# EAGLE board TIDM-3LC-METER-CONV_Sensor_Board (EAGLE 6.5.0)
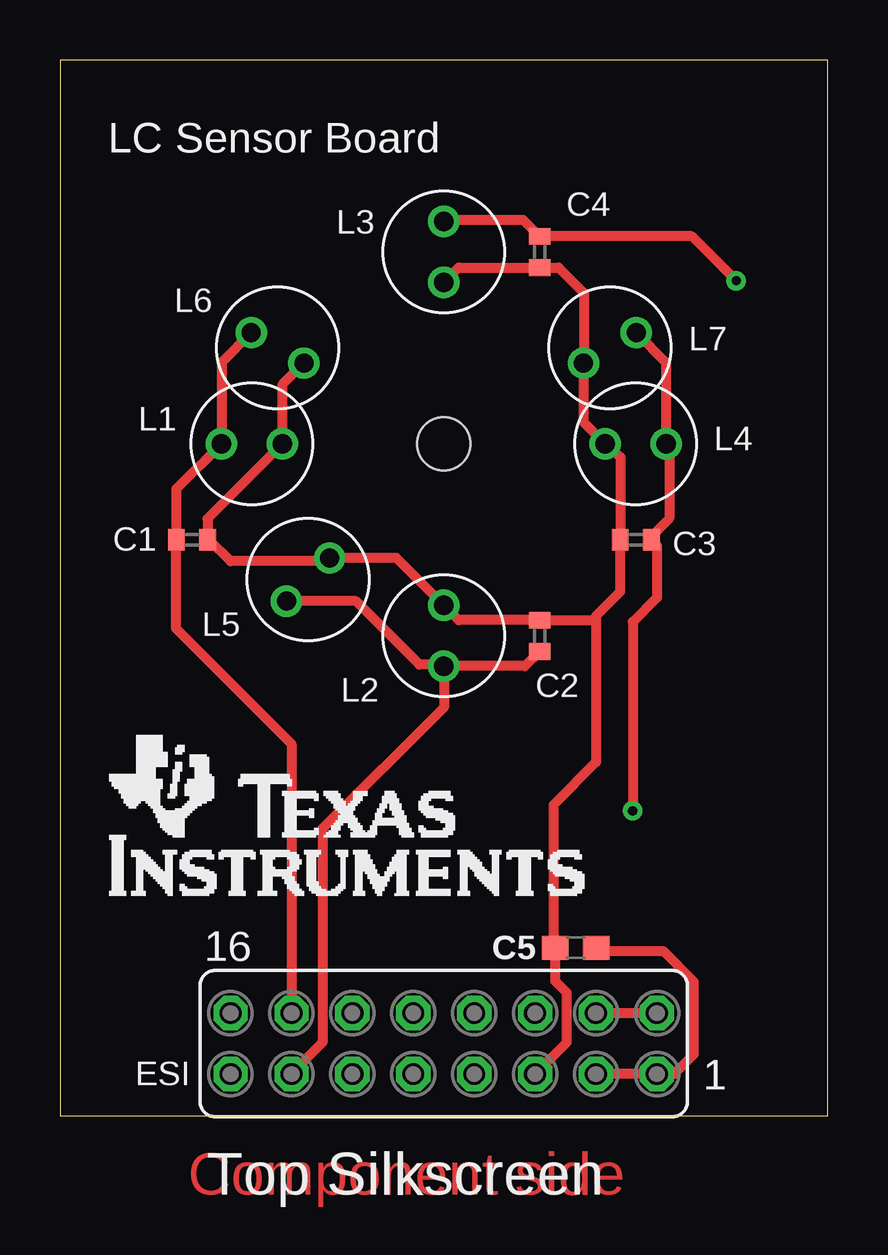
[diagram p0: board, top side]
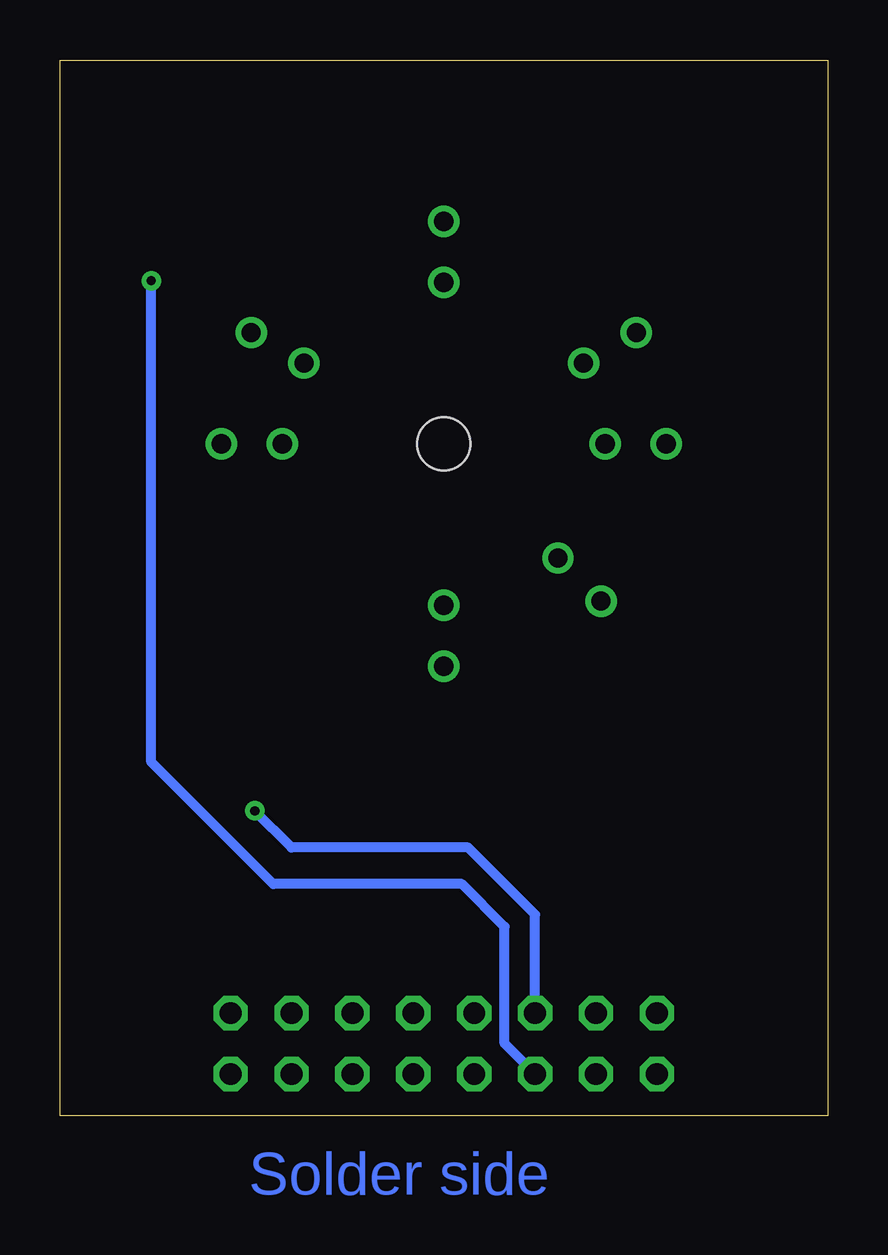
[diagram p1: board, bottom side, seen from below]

Size 32 x 44 mm. Coordinates in mm from the lower left corner, seen from the top.
Outline: 32,0 32,44 0,44 0,0 32,0
Copper layers (1*16): Top 0.035mm / dielectric 1.5mm / Bottom 0.035mm
Design rules "default": minimum track width 10mil, minimum drill 0.3mm, track to track 8mil, track to pad 8mil, pad to pad 8mil, via to via 8mil, smd to smd 8mil, copper to edge 20mil, drill to drill 8mil, minimum pad ring 10mil, minimum via ring 8mil, stop-mask expansion 4mil, vias tented up to drill 100mil, thermal gap 10mil
Holes 2.2 mm at 16,28

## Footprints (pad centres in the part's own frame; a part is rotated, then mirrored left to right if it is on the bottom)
C0402 = smd 0.7 x 0.9: 1 -0.65,0; 2 0.65,0
C0603 = smd 1.1 x 1: 1 -0.85,0; 2 0.85,0
FE08-2 = drill 0.914 octagon: 1 -8.89,1.27; 2 -8.89,-1.27; 3 -6.35,1.27; 4 -6.35,-1.27; 5 -3.81,1.27; 6 -3.81,-1.27; 7 -1.27,1.27; 8 -1.27,-1.27; 9 1.27,1.27; 10 1.27,-1.27; 11 3.81,1.27; 12 3.81,-1.27; 13 6.35,1.27; 14 6.35,-1.27; 15 8.89,1.27; 16 8.89,-1.27
0204/7 = drill 0.8: 1 -1.27,0; 2 1.27,0

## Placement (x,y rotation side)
C1  220pF  [C0402]  5.5,24 180 top
C2  220pF  [C0402]  20,20 270 top
C3  DNP  [C0402]  24,24 0 top
C4  DNP  [C0402]  20,36 90 top
C5  470nF  [C0603]  21.5,7 0 top
ESI  [FE08-2]  16,3 180 top
L1  470uH  [0204/7]  8,28 180 top
L2  470uH  [0204/7]  16,20 270 top
L3  DNP  [0204/7]  16,36 90 top
L4  DNP  [0204/7]  24,28 0 top
L5  DNP  [0204/7]  10.34,22.34 225 top
L6  DNP  [0204/7]  9.07,32 150 top
L7  DNP  [0204/7]  22.93,32 30 top
U$1  TI-LOGO-SMALL  [TI-LOGO-4]  2,9 0 top

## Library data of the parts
C1-C5 = rcl
ESI = con-lsta; OC_FARNELL: unknown; OC_NEWARK: unknown
L1-L7 = Sensor LR
U$1 = texas-logo

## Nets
ESICH0/ESITEST0: C1.2 ESI.14 L1.2 L6.2
ESICH1/ESITEST1: C2.2 ESI.13 L2.2 L5.2
ESICH2/ESITEST2: C3.2 ESI.12 L4.2 L7.2
ESICH3/ESITEST3: C4.2 ESI.11 L3.2
ESICI: ESI.6
ESICI0: ESI.10
ESICI1: ESI.9
ESICI2: ESI.8
ESICI3: ESI.7
ESICOM: C1.1 C2.1 C3.1 C4.1 C5.1 ESI.5 L1.1 L2.1 L3.1 L4.1 L5.1 L6.1 L7.1
ESITEST4: ESI.16
GND: C5.2 ESI.1 ESI.3
VCC_IO: ESI.2 ESI.4

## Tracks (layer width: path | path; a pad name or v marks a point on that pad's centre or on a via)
ESICH0/ESITEST0
  Top 0.406: L6.2 6.73,31.39 L1.2 4.85,26.12 C1.2 4.83,23.98 4.83,20.32 9.65,15.5 ESI.14
ESICH1/ESITEST1
  Top 0.406: C2.2 19.38,18.73 L2.2 15.93,18.8 | 15.93,18.8 14.99,18.8 12.34,21.45 L5.2 | 15.93,18.8 16,18.8 16,17.02 10.95,11.96 10.95,3.1 10.95,3.05 ESI.13
ESICH2/ESITEST2  (via drill 0.38 pad 0.81)
  Top 0.406: L7.2 25.27,31.39 L4.2 25.4,27.87 25.4,24.89 24.65,24.14 C3.2 24.89,23.76 24.89,21.59 23.88,20.57 23.88,12.95 v23.88,12.7
  Bottom 0.406: ESI.12 12.19,8.38 14.99,11.18 22.35,11.18 v23.88,12.7
ESICH3/ESITEST3  (via drill 0.38 pad 0.81)
  Top 0.406: L3.2 16.07,37.34 19.3,37.34 C4.2 26.34,36.65 v28.19,34.8
  Bottom 0.406: ESI.11 13.46,3 13.46,7.87 15.24,9.65 23.11,9.65 28.19,14.73 v28.19,34.8
ESICOM
  Top 0.406: ESI.5 21.12,3.04 21.12,5.12 20.65,5.6 C5.1 20.57,7.08 20.57,12.95 22.35,14.73 22.35,20.57 | L3.1 16.62,35.35 C4.1 20.78,35.35 21.84,34.29 21.84,31.38 L7.1 21.83,28.9 L4.1 22.8,28 23.37,27.43 23.37,24.02 C3.1 23.35,21.83 22.35,20.83 22.35,20.57 | 22.35,20.57 22.28,20.65 C2.1 16.62,20.65 L2.1 14.03,23.24 L5.1 11.11,23.11 7.11,23.11 6.23,24 C1.1 6.15,24.88 L1.1 9.27,30.46 L6.1
GND
  Top 0.406: ESI.3 ESI.1 25.61,1.73 26.42,2.54 26.42,5.59 25.15,6.86 22.49,6.86 C5.2
VCC_IO
  Top 0.406: ESI.2 ESI.4

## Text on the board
Top: Component side
Bottom: Solder side
tPlace: LC Sensor Board | Top Silkscreen
tStop: Top Mask
bStop: Bottom Mask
